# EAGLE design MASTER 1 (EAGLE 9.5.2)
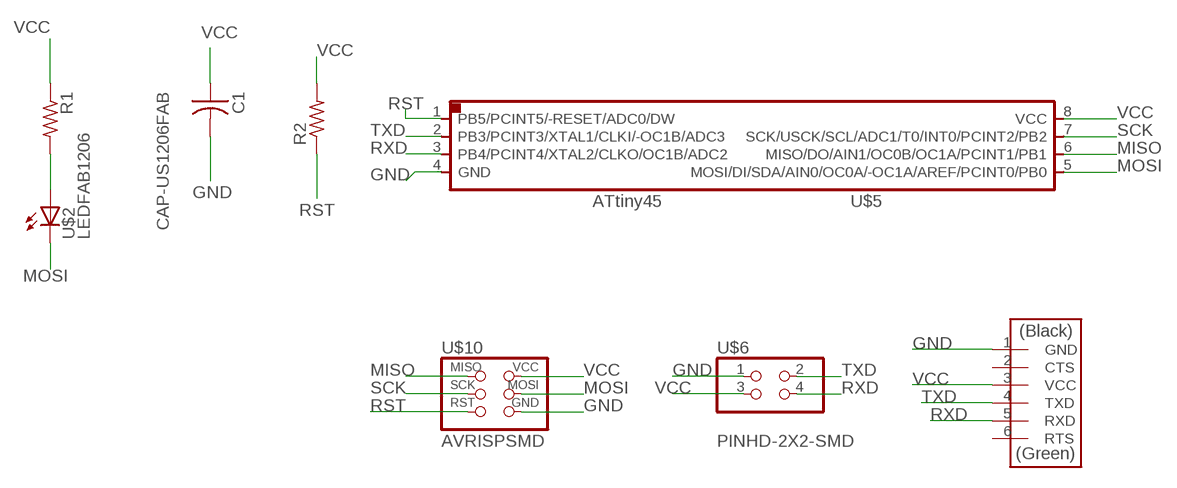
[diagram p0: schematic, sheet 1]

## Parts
C1  CAP-US1206FAB  [C1206FAB]
R1  RES-US1206FAB  [R1206FAB]
R2  RES-US1206FAB  [R1206FAB]
U$2  LEDFAB1206  [LED1206FAB]
U$3  FTDI-SMD-HEADER  [1X06SMD]
U$5  ATTINY45SI  [SOIC8]
U$6  PINHD-2X2-SMD  [2X02SMD]
U$10  AVRISPSMD  [2X03SMD]

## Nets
GND: C1.2 U$3.1(GND) U$5.4(GND) U$6.1 U$10.6(GND)
MISO: U$5.6(MISO/DO/AIN1/OC0B/OC1A/PCINT1/PB1) U$10.1(MISO)
MOSI: U$2.2(C) U$5.5(MOSI/DI/SDA/AIN0/OC0A/-OC1A/AREF/PCINT0/PB0) U$10.4(MOSI)
N$2: R1.2 U$2.1(A)
RST: R2.1 U$5.1(PB5/PCINT5/-RESET/ADC0/DW) U$10.5(RST)
RXD: U$3.5(RXD) U$5.3(PB4/PCINT4/XTAL2/CLKO/OC1B/ADC2) U$6.4
SCK: U$5.7(SCK/USCK/SCL/ADC1/T0/INT0/PCINT2/PB2) U$10.3(SCK)
TXD: U$3.4(TXD) U$5.2(PB3/PCINT3/XTAL1/CLKI/-OC1B/ADC3) U$6.2
VCC: C1.1 R1.1 R2.2 U$3.3(VCC) U$5.8(VCC) U$6.3 U$10.2(VCC)
Unconnected: U$3.2(CTS) U$3.6(RTS)

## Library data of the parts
C1 = eagle_fab:CAP-US
R1 R2 = eagle_fab:RES-US: Resistor (US Symbol)
U$2 = eagle_fab:LED: LED
U$3 = eagle_fab:FTDI-SMD-HEADER
U$5 = eagle_fab:ATTINY45
U$6 = eagle_fab:PINHD-2X2-SMD
U$10 = eagle_fab:AVRISP

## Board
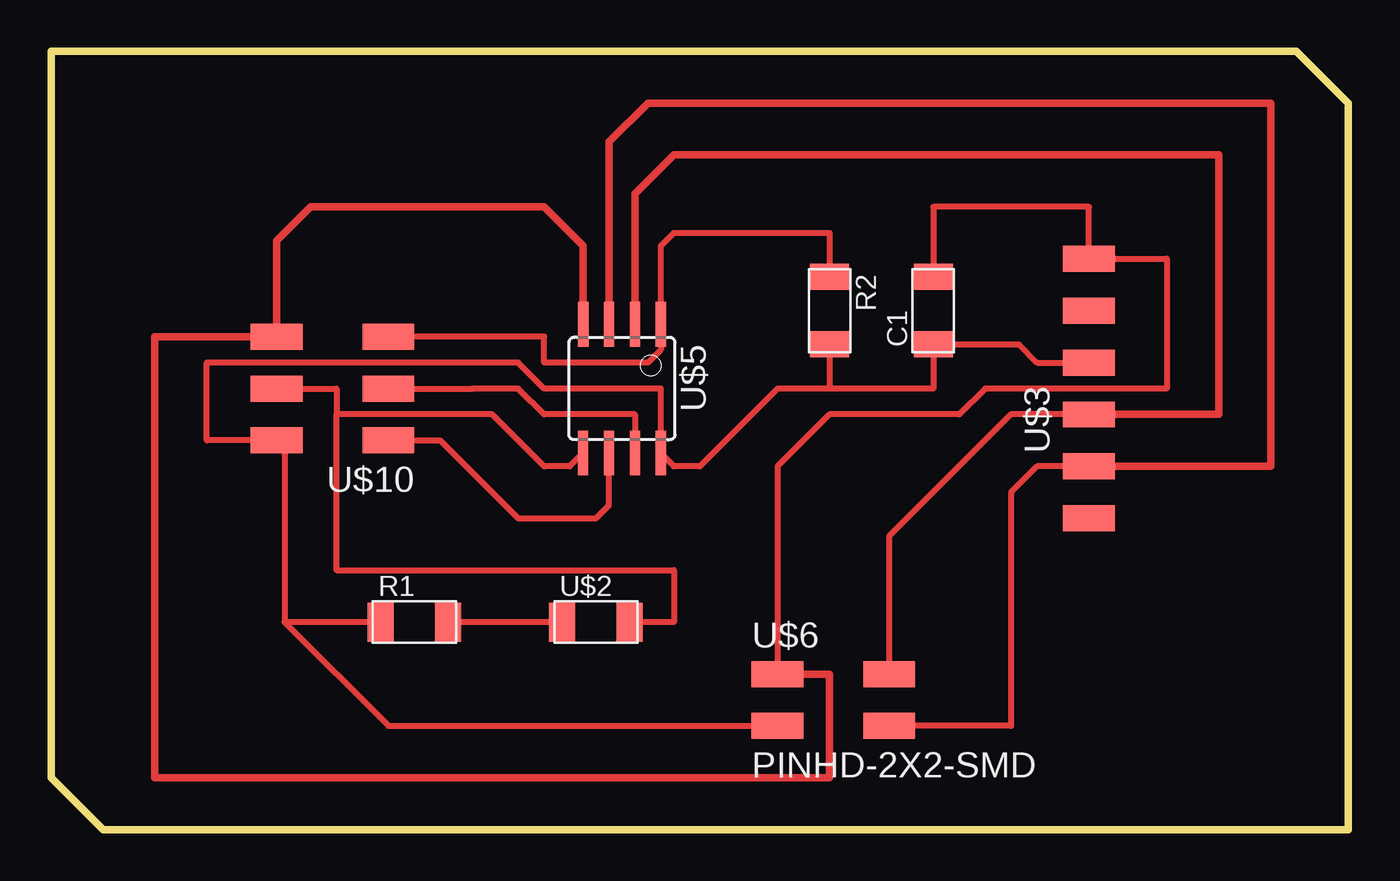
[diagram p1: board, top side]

Size 63.5 x 38.1 mm. Coordinates in mm from the lower left corner, seen from the top.
Outline: 2.54,38.1 5.08,38.1 60.96,38.1 63.5,35.56 63.5,0 2.54,0 0,2.54 0,38.1 2.54,38.1
Copper layers (1*16): Top 0.035mm / dielectric 1.5mm / Bottom 0.035mm
Design rules "default": minimum track width 6mil, minimum drill 0.35mm, track to track 6mil, track to pad 6mil, pad to pad 6mil, via to via 6mil, smd to smd 6mil, copper to edge 40mil, drill to drill 6mil, minimum pad ring 10mil, minimum via ring 8mil, stop-mask expansion 4mil, vias tented up to drill 0mil, thermal gap 10mil

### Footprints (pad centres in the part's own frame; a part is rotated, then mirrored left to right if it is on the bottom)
C1206FAB = smd 1.27 x 1.905: 1 -1.651,0; 2 1.651,0
R1206FAB = smd 1.27 x 1.905: 1 -1.651,0; 2 1.651,0
LED1206FAB = smd 1.27 x 1.905: 1 -1.651,0; 2 1.651,0
1X06SMD = smd 2.54 x 1.27: 1 0,6.35; 2 0,3.81; 3 0,1.27; 4 0,-1.27; 5 0,-3.81; 6 0,-6.35
SOIC8 = smd 0.5 x 2.2: 1 -1.905,-3.154; 2 -0.645,-3.154; 3 0.625,-3.154; 4 1.895,-3.154; 5 1.905,3.154; 6 0.635,3.154; 7 -0.635,3.154; 8 -1.905,3.154
2X02SMD = smd 2.54 x 1.27: 1 -2.54,1.27; 2 2.92,1.27; 3 -2.54,-1.27; 4 2.92,-1.27
2X03SMD = smd 2.54 x 1.27: 1 -2.54,2.54; 2 2.92,2.54; 3 -2.54,0; 4 2.92,0; 5 -2.54,-2.54; 6 2.92,-2.54

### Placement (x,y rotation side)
C1  43.18,25.4 90 top
R1  17.78,10.16 0 top
R2  38.1,25.4 270 top
U$2  26.67,10.16 0 top
U$3  50.8,21.59 0 top
U$5  27.94,21.59 180 top
U$6  38.1,6.35 0 top
U$10  13.97,21.59 180 top

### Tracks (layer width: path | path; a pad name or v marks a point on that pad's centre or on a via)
GND
  Top 0.152: 26.04,25.4 U$5.4
  Top 0.305: U$6.1 35.56,17.78 38.1,20.32 44.45,20.32 45.72,21.59 54.61,21.59 54.61,27.94 U$3.1 50.8,30.48 43.18,30.48 C1.2
  Top 0.356: U$5.4 26.04,28.57 24.13,30.48 12.7,30.48 11.05,28.83 U$10.6 5.08,24.13 5.08,2.54 38.1,2.54 38.1,7.62 U$6.1
MISO
  Top 0.305: U$10.1 19.05,19.05 22.86,15.24 26.67,15.24 27.3,15.87 U$5.6
MOSI
  Top 0.305: U$10.4 13.97,21.59 13.97,20.32 | U$5.5 25.38,17.78 24.13,17.78 21.59,20.32 13.97,20.32 | 13.97,20.32 13.97,12.7 30.48,12.7 30.48,10.16 U$2.2
N$2
  Top 0.305: U$2.1 R1.2
RST
  Top 0.305: U$10.5 24.13,24.13 24.13,22.86 29.21,22.86 29.85,23.5 U$5.1 29.85,28.57 30.48,29.21 38.1,29.21 R2.1
RXD
  Top 0.152: 40.64,5.08 U$6.4
  Top 0.305: U$3.5 48.26,17.78 46.99,16.51 46.99,5.08 40.64,5.08
  Top 0.356: U$5.3 27.32,33.66 29.21,35.56 59.69,35.56 59.69,17.78 U$3.5
SCK
  Top 0.305: U$5.7 28.57,20.32 24.13,20.32 22.86,21.59 20.62,21.59 U$10.3
TXD
  Top 0.305: U$3.4 46.99,20.32 41.02,14.35 U$6.2
  Top 0.356: U$5.2 28.58,31.12 30.48,33.02 57.15,33.02 57.15,20.32 U$3.4
VCC
  Top 0.305: U$3.3 48.26,22.86 47.37,23.75 C1.1 43.18,21.59 38.1,21.59 | 38.1,21.59 35.56,21.59 31.75,17.78 30.48,17.78 29.85,18.41 U$5.8 29.85,21.59 24.13,21.59 22.86,22.86 7.62,22.86 7.62,19.05 U$10.2 11.43,18.67 11.43,10.16 | R2.2 38.1,21.59 | R1.1 11.43,10.16 | 11.43,10.16 16.51,5.08 U$6.3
